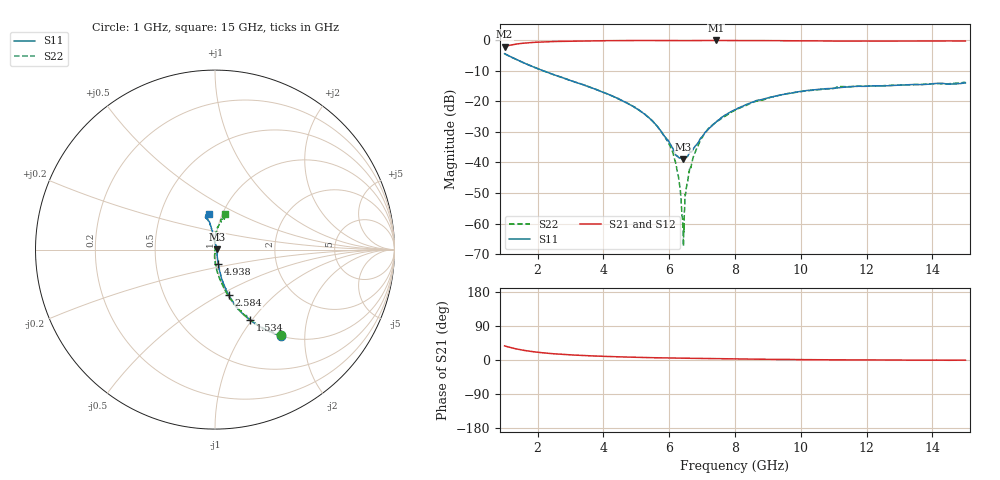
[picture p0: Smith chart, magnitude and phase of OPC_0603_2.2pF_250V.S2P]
! FILE NAME
! DATE 08/20/2012  10:21
! CORRECTED  DATA
# GHz  S  MA  R  50.00
!  FREQ  S11M  S11A  S21M  S21A  S12M  S12A  S22M  S22A
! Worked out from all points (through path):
!   1601 points, 1 GHz to 15 GHz, reference 50 ohm
!   highest |S21| = -0.05 dB at 7.423 GHz (marker M1); lowest = -2.0 dB at 1 GHz (marker M2)
!   group delay of S21, straight-line fit = 4.6 ps
!   lowest |S11| = -39.0 dB at 6.434 GHz (marker M3), VSWR 1.02, Z = 51.1 + j0.273 ohm
!   |S11| at or under -10 dB: 2.179 GHz to end of sweep
!   |S22| runs from -67.4 to -4.4 dB; largest |S21 - S12| = 0.0092
!   S11 on the Smith chart (normalised r, x): 1 GHz: 1.01, -1.52; 1.534 GHz: 1.01, -0.98; 2.584 GHz: 1.02, -0.55; 4.938 GHz: 1.02, -0.16; 15 GHz: 0.86, +0.36
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1  0.6036 -52.5  0.7904 37.3  0.7896 37.3  0.6036 -52.2
1.53375  0.4383 -63.4  0.8926 26.2  0.8918 26.2  0.4381 -63.2
2.58375  0.2635 -73.1  0.9577 15.9  0.9571 15.8  0.2632 -74.0
3.33625  0.1919 -76.1  0.9754 12.1  0.9743 12.0  0.1914 -78.7
4.9375  0.08074 -76.8  0.9916 7.3  0.9907 7.2  0.08135 -88.2
5.6725  0.03677 -71.4  0.993 5.7  0.9927 5.7  0.03693 -93.8
5.9875  0.02222 -55.2  0.9909 5.2  0.9901 5.2  0.0206 -93.6
6.13625  0.01574 -43.7  0.9904 5.0  0.9899 5.0  0.01267 -96.8
6.2675  0.01244 -20.5  0.9897 4.8  0.9888 4.8  0.006382 -90.9
6.38125  0.01148 2.7  0.9889 4.7  0.9883 4.7  0.00162 -72.7
6.43375  0.01127 13.7  0.9881 4.7  0.9878 4.6  0.0004266 23.5
6.48625  0.01193 21.7  0.9891 4.6  0.9869 4.8  0.002994 78.1
6.53  0.01223 30.1  0.9887 4.6  0.9882 4.5  0.004105 79.0
6.57375  0.01295 38.9  0.989 4.6  0.9889 4.5  0.005388 87.6
6.775  0.01792 65.0  0.9906 4.4  0.9903 4.3  0.01405 93.9
7.08125  0.03056 85.3  0.9922 4.0  0.9914 3.9  0.03049 93.9
7.4225  0.04574 93.3  0.9943 3.5  0.9924 3.4  0.04572 90.2
8  0.07321 96.9  0.9914 2.8  0.9901 2.8  0.07146 89.7
9.12  0.1184 99.3  0.9861 1.7  0.9851 1.7  0.1182 84.0
10.33625  0.1536 101.1  0.9799 0.7  0.9787 0.6  0.1514 78.2
12.6725  0.18 105.8  0.9671 -0.0  0.9667 -0.1  0.1819 73.5
15  0.2008 100.4  0.9765 -0.3  0.9756 -0.3  0.2064 74.7
